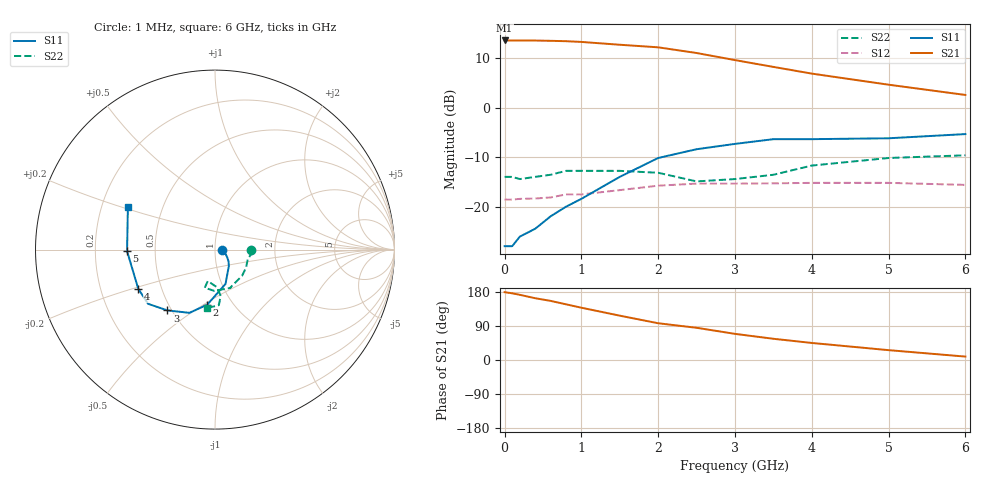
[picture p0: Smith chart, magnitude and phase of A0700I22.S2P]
!  MSA-0700 S AND NOISE PARAMETERS
!  Id=22mA  LAST UPDATED 07-27-92
# ghz s ma r 50
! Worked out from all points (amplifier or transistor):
!   15 points, 1 MHz to 6 GHz, reference 50 ohm
!   highest |S21| = 13.5 dB at 1 MHz (marker M1)
!   |S21| within 3 dB of that: start of sweep to 2.664 GHz
!   unconditionally stable (mu >= 1): start of sweep to 1.591 GHz; 3.484 GHz to end of sweep
!   at 200 MHz: K = 1.14, MAG = 13.7 dB, |S12| = -18.4 dB
!   at 1.5 GHz: K = 1.01, MAG = 13.9 dB, |S12| = -16.7 dB
!   at 6 GHz: K = 1.38, MAG = 5.4 dB, |S12| = -15.6 dB
!   lowest NFmin = 4.30 dB at 100 MHz
!   S11 on the Smith chart (normalised r, x): 1 MHz: 1.08, -0.00; 2 GHz: 0.76, -0.52; 3 GHz: 0.48, -0.40; 4 GHz: 0.37, -0.21; 5 GHz: 0.34, -0.01; 6 GHz: 0.31, +0.21
0.001  0.04 -1.0  4.75 179.0  0.118 0.0  0.2 -1.0
0.1  0.04 -5.0  4.75 176.0  0.118 2.0  0.2 -9.0
0.2  0.05 -8.0  4.74 172.0  0.12 3.0  0.19 -16.0
0.4  0.06 -19.0  4.74 163.0  0.121 7.0  0.2 -30.0
0.6  0.08 -32.0  4.71 156.0  0.124 9.0  0.21 -44.0
0.8  0.1 -41.0  4.67 147.0  0.133 12.0  0.23 -69.0
1  0.12 -50.0  4.59 138.0  0.133 13.0  0.23 -68.0
1.5  0.2 -73.0  4.3 117.0  0.147 17.0  0.23 -91.0
2  0.31 -98.0  4.05 97.0  0.163 17.0  0.22 -105.0
2.5  0.38 -112.0  3.55 85.0  0.171 18.0  0.18 -103.0
3  0.43 -128.0  3.01 69.0  0.171 17.0  0.19 -96.0
3.5  0.48 -141.0  2.57 56.0  0.172 17.0  0.21 -87.0
4  0.48 -153.0  2.2 45.0  0.174 14.0  0.26 -83.0
5  0.49 -179.0  1.7 26.0  0.174 12.0  0.31 -86.0
6  0.54 154.0  1.34 9.0  0.166 13.0  0.33 -98.0
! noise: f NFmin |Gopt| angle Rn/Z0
0.1  4.3  0.05  3  0.6
0.5  4.4  0.05  15  0.59
1  4.5  0.04  38  0.58
2  5  0.03  137  0.56
